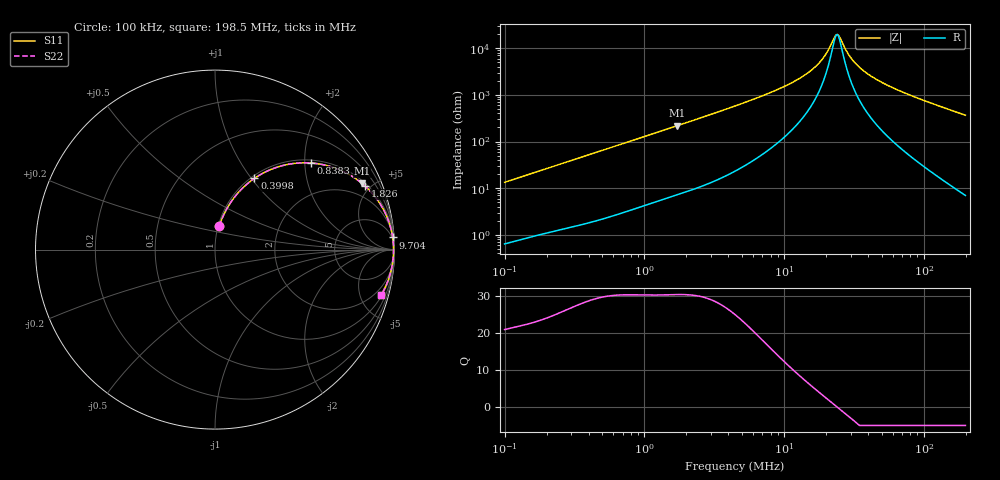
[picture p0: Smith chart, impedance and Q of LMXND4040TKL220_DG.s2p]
! LMXND4040TKL220_DG  S-PARAMETER MODEL  ( General Type )
! Model Generated by TAIYO YUDEN Corporation (http://www.ty-top.com)
! Version 1.0
! TAIYO YUDEN Control No. 191023NI43SB-FBB
! Copyright(c) 2019 TAIYO YUDEN CO.,LTD. All Rights Reserved.
! Product Description (link to TY-COMPAS)
! https://ds.yuden.co.jp/TYCOMPAS/or/detail?pn=LMXND4040TKL220MDG&u=M
! Products Name : Inductors
! Characteristics :
!  Inductance : 22 uH , SRF(min) : 15 MHz , DC Resistance(max) : 0.348 Ohm
!  Rated Current : Saturation :900 mA , Temp Rise : 720 mA
!  Case Size : 4.0 x 4.0 / 0.157 x 0.157 [mm/inch] , Thickness : 1.8 / 0.071 [mm/inch]
!  (Conditions: Temperature = 25 degC , DC Bias Current/Voltage = 0A / 0V)
! External Node Assignments :
!  1  o---GGG---o  2
! GND o---------o GND
! Frequency Range : 0.1MHz  -  198.534594MHz  [ 402 STEP ]
# MHz S RI R 50
! Freq[MHz].  S11 Real  S11 Imag  S21 Real  S21 Imag  S12 Real  S12 Imag  S22 Real  S22 Imag
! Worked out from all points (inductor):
!   401 points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, 100 kHz to 198.5 MHz, reference 50 ohm
!   read as one part in series: L = 21.1 uH near 103.9 kHz
!   highest Q = 30.3 at 1.725 MHz (marker M1), where L = 20.2 uH
!   self-resonance near 23.68 MHz
!   S11 on the Smith chart (normalised r, x): 100 kHz: 1.01, +0.27; 399.8 kHz: 1.04, +1.04; 838.3 kHz: 1.07, +2.15; 1.826 MHz: 1.15, +4.63; 9.704 MHz: 3, +29; 198.5 MHz: 1.14, -7.33
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0.1  0.0236 0.1296  0.9764 -0.1296  0.9764 -0.1296  0.0236 0.1296
0.205728  0.0769 0.2465  0.9231 -0.2465  0.9231 -0.2465  0.0769 0.2465
0.356769  0.1853 0.371  0.8147 -0.371  0.8147 -0.371  0.1853 0.371
0.399811  0.2196 0.3969  0.7804 -0.3969  0.7804 -0.3969  0.2196 0.3969
0.83829  0.5343 0.4825  0.4657 -0.4825  0.4657 -0.4825  0.5343 0.4825
1.272844  0.7176 0.4339  0.2824 -0.4339  0.2824 -0.4339  0.7176 0.4339
1.724601  0.8192 0.3687  0.1808 -0.3687  0.1808 -0.3687  0.8192 0.3687
1.82567  0.8348 0.3553  0.1652 -0.3553  0.1652 -0.3553  0.8348 0.3553
4.541117  0.9657 0.1628  0.0343 -0.1628  0.0343 -0.1628  0.9657 0.1628
9.7039  0.9899 0.068  0.0101 -0.068  0.0101 -0.068  0.9899 0.068
12.90076  0.9929 0.0436  0.00713 -0.0436  0.00713 -0.0436  0.9929 0.0436
15.89665  0.9941 0.0279  0.00592 -0.0279  0.00592 -0.0279  0.9941 0.0279
18.85849  0.9947 0.016  0.00534 -0.016  0.00534 -0.016  0.9947 0.016
22.80095  0.9949 0.00331  0.00506 -0.00331  0.00506 -0.00331  0.9949 0.00331
24.13719  0.995 -0.000457  0.00504 0.000457  0.00504 0.000457  0.995 -0.000457
25.07124  0.995 -0.00297  0.00505 0.00297  0.00505 0.00297  0.995 -0.00297
29.18318  0.9948 -0.0131  0.00519 0.0131  0.00519 0.0131  0.9948 -0.0131
33.96951  0.9944 -0.0235  0.00557 0.0235  0.00557 0.0235  0.9944 -0.0235
41.85813  0.9935 -0.0388  0.00652 0.0388  0.00652 0.0388  0.9935 -0.0388
56.71438  0.9909 -0.0641  0.00914 0.0641  0.00914 0.0641  0.9909 -0.0641
98.35271  0.9788 -0.1257  0.0212 0.1257  0.0212 0.1257  0.9788 -0.1257
198.5346  0.9265 -0.2515  0.0735 0.2515  0.0735 0.2515  0.9265 -0.2515
